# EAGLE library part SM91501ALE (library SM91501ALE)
Audio Transformers / Signal Transformers BMS xformer 2-Ch 1600V AECQ +125 C Source: Datasheet
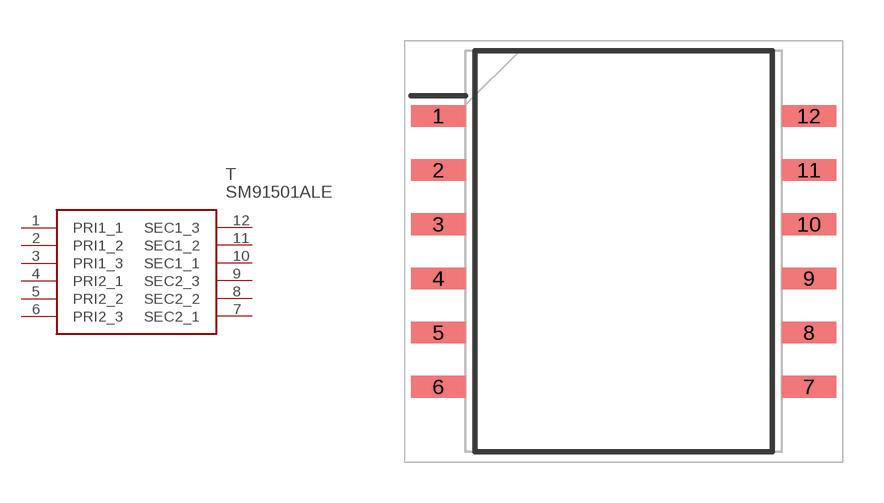
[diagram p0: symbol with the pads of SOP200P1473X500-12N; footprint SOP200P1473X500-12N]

Designator prefix T

## SM91501ALE (Description: Audio Transformers / Signal Transformers BMS xformer 2-Ch 1600V AECQ +125 C; Height: 5mm; Manufacturer_Name: Bourns; Manufacturer_Part_Number: SM91501ALE; Mouser_Part_Number: 652-SM91501ALE; Mouser_Price-Stock: https://www.mouser.co.uk/ProductDetail/Bourns/SM91501ALE?qs=qSfuJ%252Bfl%2Fd67nNHsx2b1iA%3D%3D)  [SOP200P1473X500-12N]
1  PRI1_1
2  PRI1_2
3  PRI1_3
4  PRI2_1
5  PRI2_2
6  PRI2_3
7  SEC2_1
8  SEC2_2
9  SEC2_3
10  SEC1_1
11  SEC1_2
12  SEC1_3

## Footprint SOP200P1473X500-12N (pad centres in mm)
12-PIN SMD/SMT
smd 2.01 x 0.8: 1 -6.845,5; 2 -6.845,3; 3 -6.845,1; 4 -6.845,-1; 5 -6.845,-3; 6 -6.845,-5; 7 6.845,-5; 8 6.845,-3; 9 6.845,-1; 10 6.845,1; 11 6.845,3; 12 6.845,5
